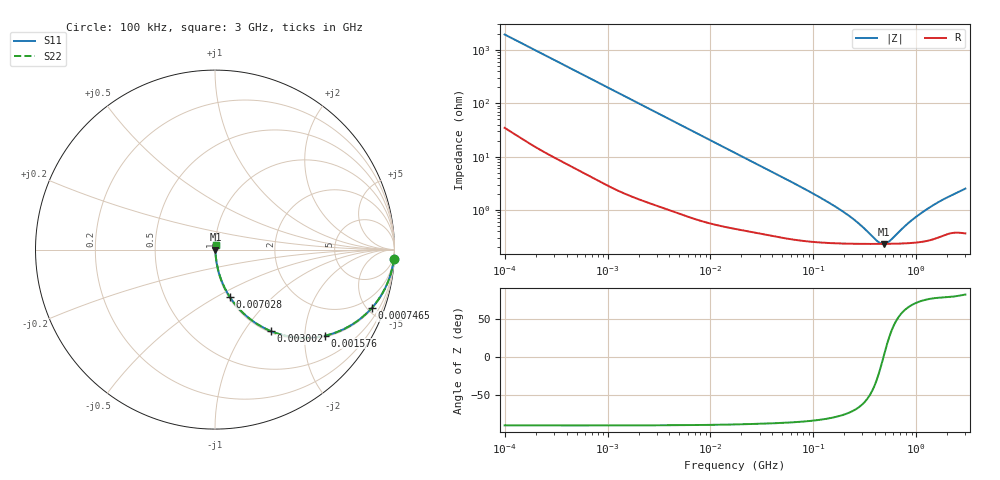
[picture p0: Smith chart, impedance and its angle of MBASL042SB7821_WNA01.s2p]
! MBASL042SB7821_WNA01  S-PARAMETER MODEL  ( Standard Model )
! Model Generated by TAIYO YUDEN Corporation (https://www.yuden.co.jp/en/)
! Version 1.0
! TAIYO YUDEN Control No. 250312
! Copyright(c) 2025 TAIYO YUDEN CO.,LTD. All Rights Reserved.
! Product Description (link to TY-COMPAS)
! https://ds.yuden.co.jp/TYCOMPAS/or/detail?pn=MBASL042SB7821KWNA01&u=M
! Products Name : Multilayer Ceramic Capacitors
! Characteristics :
!  Capacitance : 820 [pF] , Rated Voltage : 10 [V] , TCC : X7R
!  Case Size : 0.4 x 0.2 / 0.016 x 0.008 [mm/inch] , Thickness : 0.2 / 0.008 [mm/inch]
!  (Conditions: Temperature = 25 [degC] , DC Bias Voltage = 0 [V])
! External Node Assignments :
!  1  o---| |---o  2
! GND o---------o GND
! Frequency Range : 100kHz  -  3GHz  [ 401 STEP ]
# MHZ S RI R 50
! Freq[MHz].  S11 Real  S11 Imag  S21 Real  S21 Imag  S12 Real  S12 Imag  S22 Real  S22 Imag
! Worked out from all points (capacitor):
!   401 points, 100 kHz to 3 GHz, reference 50 ohm
!   read as one part in series: C = 814 pF near 105.3 kHz
!   lowest |Z| = 232 mohm at 481.3 MHz (marker M1)
!   series resonance near 479.6 MHz, so ESL is about 140 pH
!   S11 on the Smith chart (normalised r, x): 100 kHz: 2, -39; 746.5 kHz: 1.08, -5.32; 1.576 MHz: 1.04, -2.53; 3.002 MHz: 1.02, -1.34; 7.028 MHz: 1.01, -0.58; 3 GHz: 1.01, +0.05
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0.1  0.9965 -0.0511  0.00353 0.0511  0.00353 0.0511  0.9965 -0.0511
0.252895  0.9819 -0.126  0.0181 0.126  0.0181 0.126  0.9819 -0.126
0.562235  0.9221 -0.2607  0.0779 0.2607  0.0779 0.2607  0.9221 -0.2607
0.746515  0.8725 -0.3264  0.1275 0.3264  0.1275 0.3264  0.8725 -0.3264
1.070873  0.7722 -0.4123  0.2278 0.4123  0.2278 0.4123  0.7722 -0.4123
1.576268  0.6141 -0.4793  0.3859 0.4793  0.3859 0.4793  0.6141 -0.4793
2.147551  0.4651 -0.4907  0.5349 0.4907  0.5349 0.4907  0.4651 -0.4907
3.002272  0.3118 -0.4543  0.6882 0.4543  0.6882 0.4543  0.3118 -0.4543
3.161081  0.2908 -0.4451  0.7092 0.4451  0.7092 0.4451  0.2908 -0.4451
4.652942  0.1629 -0.3592  0.8371 0.3592  0.8371 0.3592  0.1629 -0.3592
7.027689  0.0817 -0.2624  0.9183 0.2624  0.9183 0.2624  0.0817 -0.2624
17.7727  0.0172 -0.1122  0.9828 0.1122  0.9828 0.1122  0.0172 -0.1122
97.38194  0.00294 -0.0205  0.9971 0.0205  0.9971 0.0205  0.00294 -0.0205
210.9903  0.0024 -0.00798  0.9976 0.00798  0.9976 0.00798  0.0024 -0.00798
287.4592  0.00233 -0.00466  0.9977 0.00466  0.9977 0.00466  0.00233 -0.00466
412.3589  0.00231 -0.00132  0.9977 0.00132  0.9977 0.00132  0.00231 -0.00132
481.3181  0.00231 3.25e-05  0.9977 -3.25e-05  0.9977 -3.25e-05  0.00231 3.25e-05
547.5153  0.00232 0.00116  0.9977 -0.00116  0.9977 -0.00116  0.00232 0.00116
826.9535  0.0024 0.00501  0.9976 -0.00501  0.9976 -0.00501  0.0024 0.00501
1186.261  0.00264 0.00909  0.9974 -0.00909  0.9974 -0.00909  0.00264 0.00909
1791.7  0.00347 0.015  0.9965 -0.015  0.9965 -0.015  0.00347 0.015
3000  0.00424 0.0247  0.9958 -0.0247  0.9958 -0.0247  0.00424 0.0247
